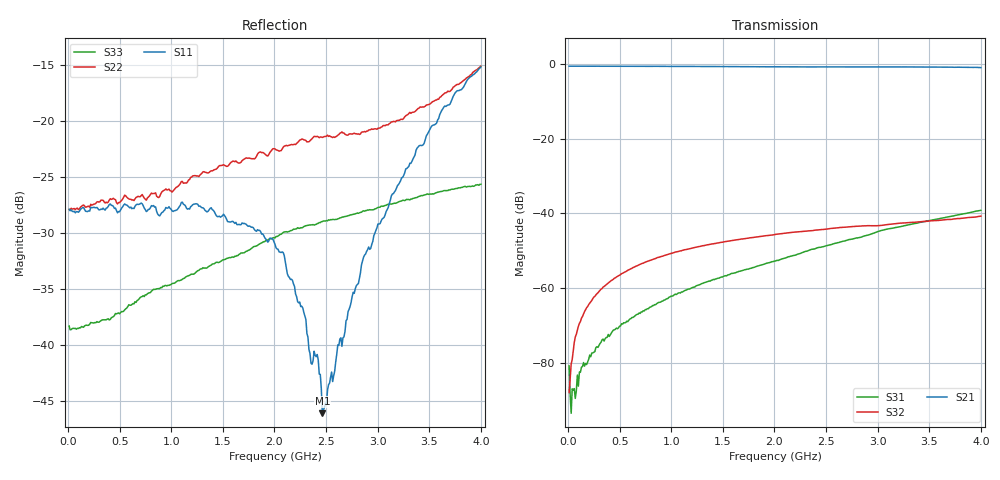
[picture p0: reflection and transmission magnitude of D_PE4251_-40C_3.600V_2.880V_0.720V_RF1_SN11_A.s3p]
! Device ID: PE4251_SoldCshunt_081809
! Dir: c:\Test Bench Repositories\Bench_Software_CVI_Version_8\trunk\PSC 4Port_VNA Bench\datalog\4250\TEST\PE4251_SoldCshunt_081809\-40C\3p600000\RF1
! Serial: 11
! Insertion: A
! Temp: -40C
! VDD: 3.600
! Control_Hi: 80.000
! Control_Lo: 20.000
! Logic State: RF1
! Port 1: RFC
! Port 2: RF1
! Port 3: RF2
! V1 = 0.72
! V2 = 2.88
! V3 = 0.72
! IDD: 5.028610e-05
! FILE NAME
! DATE 08/18/09  20:09
! CORRECTED  DATA
#  Hz  S  RI  R  50.00
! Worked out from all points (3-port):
!   401 points, 10 MHz to 4 GHz, reference 50 ohm
!   strongest paths, dB at 10 MHz, 1.008 GHz, 2.005 GHz, 3.002 GHz, 4 GHz:
!     S21: -0.5, -0.5, -0.6, -0.7, -0.9
!     S32: -88.0, -50.7, -45.7, -43.3, -40.7
!     S31: -80.9, -62.2, -52.8, -44.8, -39.2
!   lowest |S11| = -46.1 dB at 2.464 GHz (marker M1), VSWR 1.01, Z = 50.2 - j0.468 ohm
!   |S11| at or under -10 dB: start of sweep to end of sweep
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1e7  0.0404 8.61e-05  0.9453 -0.00377  1.13e-05 2.1e-05
     0.9451 -0.0039  0.0403 0.000304  1.04e-05 6.85e-05
     2e-05 -8.78e-05  3.67e-05 -1.48e-05  0.0122 -0.000375
1.79575e8  0.0395 0.000787  0.9429 -0.0609  -1.68e-05 -0.000105
           0.9428 -0.0611  0.0414 0.000504  4.6e-05 0.000542
           -3.52e-06 -9.38e-05  4.06e-05 0.000543  0.0122 0.00159
5.287e8  0.0414 -0.00211  0.9265 -0.1742  -0.000178 -0.000269
         0.9266 -0.1742  0.0449 -0.00122  0.000158 0.00158
         -0.000189 -0.000269  0.000157 0.00157  0.0135 0.00416
1.296775e9  0.0402 -0.00846  0.8417 -0.4094  -0.00105 -0.000456
            0.844 -0.4092  0.057 -0.0133  0.000756 0.00359
            -0.00106 -0.000444  0.000756 0.00358  0.0173 0.0135
2.005e9  0.0263 -0.0102  0.722 -0.5836  -0.00226 -0.000458
         0.722 -0.5837  0.0664 -0.0353  0.00122 0.00506
         -0.00225 -0.000453  0.0012 0.00507  0.0184 0.0238
2.2843e9  0.0106 -0.0091  0.6666 -0.6434  -0.003 -0.000555
          0.6652 -0.6445  0.0645 -0.0512  0.00137 0.0056
          -0.00298 -0.000567  0.00137 0.0056  0.017 0.0292
2.46385e9  0.00166 -0.00467  0.63 -0.6785  -0.00351 -0.000501
           0.6283 -0.678  0.0616 -0.0579  0.00138 0.00591
           -0.00352 -0.000499  0.00137 0.00593  0.0156 0.032
2.86285e9  -0.018 -0.0169  0.5371 -0.7549  -0.00493 -0.000443
           0.5382 -0.7528  0.0429 -0.0785  0.0015 0.00663
           -0.00494 -0.000436  0.00151 0.00663  0.0112 0.0381
3.14215e9  -0.0363 -0.0303  0.4654 -0.7996  -0.00633 -3.37e-05
           0.4666 -0.7983  0.0224 -0.0966  0.00116 0.00714
           -0.00633 -3.92e-05  0.00118 0.00715  0.00688 0.0422
4e9  -0.1564 -0.0774  0.1845 -0.8892  -0.0108 0.00213
     0.1838 -0.887  -0.12 -0.1286  4.53e-05 0.00918
     -0.0108 0.0021  2.46e-05 0.0092  -0.0133 0.0505
